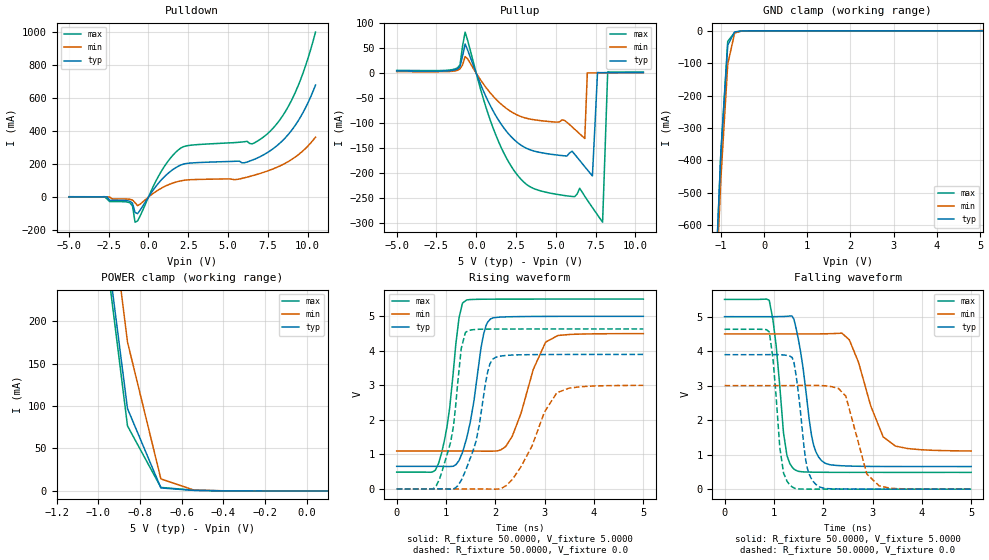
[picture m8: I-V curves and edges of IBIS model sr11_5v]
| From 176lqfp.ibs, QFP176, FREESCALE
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[Model] sr11_5v
|   Model sr11_5v
Model_type 3-state
Polarity   Non-Inverting
Enable   Active-High
Vmeas = 2.5
C_comp   4.6864pF   4.5021pF   4.9391pF
[Temperature Range]   25.0000   0.1500k   -40.0000
[Voltage Range]   5.0000V   4.5000V   5.5000V
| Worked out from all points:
|   slope of the pulldown table from 0 to 0.75 V, typ, clamps not added: 7.68 ohm
|   slope of the pullup table from 0 to 0.75 V, typ, clamps not added: 13.3 ohm
|   GND clamp passes 1 mA (typ) near -0.55 V on its own axis
|   POWER clamp passes 1 mA (typ) near -0.56 V on its own axis
|   rising waveform, R_fixture 50.0000, V_fixture 5.0000: 20-80 % time 288ps typ, 471ps min, 246ps max; typ from 0.654 V to 5 V
|   rising waveform, R_fixture 50.0000, V_fixture 0.0: 20-80 % time 346ps typ, 574ps min, 277ps max; typ from 0 V to 3.9 V
|   falling waveform, R_fixture 50.0000, V_fixture 5.0000: 20-80 % time 244ps typ, 465ps min, 194ps max; typ from 5 V to 0.656 V
|   falling waveform, R_fixture 50.0000, V_fixture 0.0: 20-80 % time 187ps typ, 340ps min, 163ps max; typ from 3.9 V to 0 V
[Pulldown]
|Voltage   I(typ)   I(min)   I(max)
-5V       1.53mA     880uA      2.56mA
-1.16V    -25.12mA   -13.09mA   -34.58mA
-1V       -37.25mA   -17.42mA   -53.52mA
-840mV    -92.5mA    -33.26mA   -151.4mA
-680mV    -99.64mA   -51.21mA   -143.5mA
920mV     115.2mA    59.46mA    173.2mA
2.04V     194.1mA    98.32mA    296.8mA
7V        243.5mA    142.5mA    347.7mA
7.96V     301.6mA    175.6mA    430.1mA
8.92V     393.8mA    222.5mA    570.8mA
9.72V     511.7mA    280.4mA    750.6mA
10.5V     676.7mA    362.1mA    997mA
[Pullup]
|Voltage   I(typ)   I(min)   I(max)
-5V       4.5mA      3.3mA      5.8mA
-1.18V    8.798mA    5.978mA    10.76mA
-700mV    58.59mA    33.39mA    82.56mA
900mV     -65.93mA   -40.08mA   -95.9mA
2.5V      -136.5mA   -82.51mA   -200.6mA
6.82V     -187.3mA   -130.8mA   -246.6mA
6.98V     -193.5mA   798uA      -254.2mA
7.3V      -205.9mA   708uA      -269.3mA
7.62V     1.458mA    738uA      -284mA
7.94V     1.26mA     764uA      -298.6mA
8.26V     1.313mA    790uA      2.953mA
10.5V     1.59mA     940uA      2.56mA
[GND_clamp]
|Voltage   I(typ)   I(min)   I(max)
-5V       -15.81A    -15.65A    -16.01A
-1.16V    -883.1mA   -945.9mA   -900.9mA
-1V       -378.6mA   -458.6mA   -378.5mA
-840mV    -44.11mA   -102.9mA   -32.53mA
-680mV    -3.439mA   -6.731mA   -5.118mA
-520mV    -530.1uA   -781.9uA   -565.8uA
-360mV    -4.994uA   -45.89uA   -1.591uA
5.08V     230.9pA    1.498mA    9.384pA
[POWER_clamp]
|Voltage   I(typ)   I(min)   I(max)
-5V       11.12A     11.24A     11.12A
-1.02V    405.3mA    491.3mA    392.9mA
-860mV    97.05mA    175.5mA    76.65mA
-700mV    3.541mA    14.18mA    4.132mA
-540mV    594.7uA    858.4uA    773.9uA
100mV     54.85pA    7.446nA    9.775pA
[Ramp]
| variable   typ   min   max
dV/dt_r  2.3380/0.3459n   1.7998/0.5424n   2.7807/0.2744n
dV/dt_f  2.6065/0.2439n   2.0359/0.4316n   3.0082/0.1867n
R_load = 50.0000
[Rising Waveform]
R_fixture= 50.0000
V_fixture= 5.0000
V_fixture_min= 4.5000
V_fixture_max= 5.5000
|time   V(typ)   V(min)   V(max)
0s        654.4mV    1.099V     486.8mV
848.8ps   654.7mV    1.099V     740.3mV
1.075ns   649.9mV    1.099V     2.351V
1.263ns   821.7mV    1.099V     4.955V
1.42ns    1.479V     1.099V     5.475V
1.761ns   4.476V     1.094V     5.495V
1.901ns   4.924V     1.093V     5.496V
2.341ns   4.989V     1.52V      5.498V
3.02ns    4.997V     4.254V     5.499V
5ns       5V         4.499V     5.5V
[Rising Waveform]
R_fixture= 50.0000
V_fixture= 0.0
V_fixture_min= 0.0
V_fixture_max= 0.0
|time   V(typ)   V(min)   V(max)
0s        5.255nV    134.1nV    18.89nV
866ps     1.096mV    102.2uV    277.4mV
1.095ns   -6.335mV   85.76uV    1.365V
1.308ns   245.5mV    166.4uV    4.065V
1.393ns   519.7mV    346uV      4.535V
1.606ns   1.371V     756uV      4.62V
1.943ns   3.754V     -6.02mV    4.631V
2.521ns   3.886V     646mV      4.633V
3.246ns   3.894V     2.785V     4.633V
5ns       3.897V     3V         4.634V
[Falling Waveform]
R_fixture= 50.0000
V_fixture= 5.0000
V_fixture_min= 4.5000
V_fixture_max= 5.5000
|time   V(typ)   V(min)   V(max)
0s        5V         4.5V       5.5V
906.8ps   5V         4.5V       5.476V
1.047ns   5.001V     4.5V       4.155V
1.195ns   5.006V     4.5V       1.636V
1.407ns   4.924V     4.5V       582.6mV
1.767ns   1.53V      4.5V       493mV
1.966ns   828.3mV    4.502V     490mV
2.529ns   669.6mV    4.332V     486.8mV
3.216ns   657.5mV    1.518V     486.8mV
5ns       655.8mV    1.107V     486.3mV
[Falling Waveform]
R_fixture= 50.0000
V_fixture= 0.0
V_fixture_min= 0.0
V_fixture_max= 0.0
|time   V(typ)   V(min)   V(max)
0s        3.898V     3.003V     4.635V
907.5ps   3.9V       3.003V     4.558V
1.121ns   3.898V     3.003V     1.203V
1.371ns   3.816V     3.003V     64.47mV
1.647ns   835.1mV    3.006V     3.644mV
1.856ns   132.7mV    3.007V     1.206mV
2.459ns   4mV        2.698V     172.8uV
2.886ns   1.486mV    436.1mV    188.6uV
3.136ns   1.02mV     95.41mV    -1.136uV
5ns       349.6uV    963.3uV    -30.4uV
